PROGRAM PickAndPlace //TF5420 PickAndPlace解决方案
VAR	
	(*抓取动作功能块（其中重要的以***标出）*)
	//轴组相关功能块
    fbAddAllAxes			                     : FB_AddAllAxes;//***将笛卡尔坐标系轴加入组
	fbGroupEnable			                     : MC_GroupEnable;//***轴组使能
	fbStop					                     : MC_GroupStop;//轴组停止
	fbUngroupAxes			                     : MC_UngroupAllAxes;//解耦轴组
	fbGroupReset			                     : MC_GroupReset;//***轴组复位
	fbGroupReadStatus		                     : MC_GroupReadStatus;//***读取轴组状态,用于报错判断
	fbGroupSetOvr			                     : MC_GroupSetOverride;//设定轴组override
    fbRemoveAllAxes                              : FB_RemoveAllAxes;//清除组中的所有轴
	
	//抓取、皮带跟随功能块
    fbMovePath				                     : MC_MovePath;//***插补动作与皮带跟随触发功能块
	fbMoveLinPrep			                     : MC_MoveLinearAbsolutePreparation;//***插补形式绝对定位
	buffer					                     : ARRAY[1..4096] OF BYTE;//插补路径点位数组
	path					                     : MC_PATH_DATA_REF(ADR(buffer), SIZEOF(buffer));
	fbTrackConveyBelt_01                         : MC_TrackConveyorBelt;//***皮带跟随功能块
	InitialObjectPos                             : ARRAY[1..4] OF MC_Lreal;//***相机读取物料点位
	
	//辅助功能块
    fbTestBeltMoveVelo                           : MC_MoveVelocity;//匀速运动
	fbTestBeltPower                              : MC_Power;//使能
    T20ms , T50ms ,TonResetDelay                 : Ton;//辅助计时器
	fbBeltReset                                  : MC_Reset;//皮带复位

   (*所用变量*)
	aTargetPos				: ARRAY[1..4] OF MC_LREAL;  //插补路径点位
	aTransitionParam		: ARRAY[1..2] OF MC_LREAL; //曲线的过渡转换参数
	MasterRefPos            : LREAL; //输料皮带当前位置
	lrDistance              : LREAL; //差值距离
    fVelFactor				: LREAL := 1.0;//速比
	nState					: INT := 0; //抓放动作Case步
    nGroupState             : UINT; //PickAndPlace轴组Case步
	bMovePrepError			: BOOL; //轴组准备报错步
	
	//轴组触发位标志位
	GroupEnable             : BOOL;	//轴组触发使能
	GroupReset				: BOOL; //轴组复位
	bpop1					: BOOL; //队列标志位
	RemoveAxes              : BOOL; //移除轴
	ReConfigAxis            : BOOL; //解耦轴组
	
	//NCI G代码回零功能块
	//NCI G代码功能块
	FB_BuildNciGroup            : CfgBuildExt3DGroup;//配置NCI通道
    FB_LoadNciProg              : ItpLoadProgEx;//加载G代码文件                 
	FB_StartGProg               : ItpStartStopEx;//启动停止
	FB_CfgReconfigGroup         : CfgReconfigGroup;//清除NCI通道
	FB_ItpResetGroup            : ItpResetEx2;//复位NCI通道
	FB_CfgReConfigAxis          : ARRAY[1..3] OF CfgReconfigAxis;//清除轴，从插补轴变回NC轴
	L_Override                  : LREAL  :=100;  //通道速比
	ProgName                    : STRING(255):='Home.nc';//G代码文件名
	Gstep                       : INT;
    uiItpState                  : UDINT; //插补通道状态返回值
	StartGProHome               : BOOL; //G代码回零触发位
	IsHoming                    : BOOL;
	
	
	
END_VAR

A_TrackConvey();//皮带跟随功能块调用
A_GroupCommand();//轴组指令
A_GProgHome();//G代码回零

CASE nState OF
0:  
	IF nGroupState=30 THEN//判断PickAndPlace轴组是否使能
	   gCurrentMaterial :=	gStmaterialNULL;//清零
	   //使用MemoryCmp来对比队列中是否有数据，有数组则允许取队列中的数组
	   IF (MEMCMP(pBuf1:= ADR(gArrayStmaterial[1]), pBuf2:=ADR(gStmaterialNULL) , n:=SIZEOF(gArrayStmaterial[1]) )<>0) THEN
		   bpop1	:=	TRUE; //标志为置位
		   nState	:=	1;			
	   END_IF
	END_IF
1:
   //若队列未在取数据，且可取标志位置位,则取
   IF NOT gbPushPopBusy AND bpop1 THEN
		  gfbPushPopStack.PopStack();
		  bpop1	:=	FALSE;
   END_IF
   //取数据，将数据赋值到变量中
   gfbPushPopStack(ArrayStmaterial:=gArrayStmaterial , PushStmaterial:= , PopStmaterial=> gCurrentMaterial, busy=>gbPushPopBusy );
  //相机发送物料坐标信息，将信息赋值到MC_TrackConveyOrBelt功能块中
   IF gCurrentMaterial.bmaterial THEN
	  InitialObjectPos[1]:=gCurrentMaterial.lrCenterX;//X轴
	  InitialObjectPos[2]:=gCurrentMaterial.lrCenterY;//Y轴
      InitialObjectPos[3]:=2;//Z轴
      InitialObjectPos[4]:=ABS(180-gCurrentMaterial.lrAngle);//C轴
	  MasterRefPos:=gCurrentMaterial.lrPhotoBeltPos;//输料皮带当前位置
      A_PreparePathPick();//调用抓取参数
	  nState := 20;
   END_IF

   
20:
   //计算输料皮带当前位置减去记录位置，当到达抓取范围内后便可抓取
   lrDistance:=BeltAxis.NcToPlc.ActPos-MasterRefPos  + InitialObjectPos[1];
   //抓取范围在X轴的-180到100之间，此单位内允许抓取
   IF lrDistance>=-180 AND lrDistance<=100  THEN
	    fbTrackConveyBelt_01.Execute :=TRUE;
	    IF fbTrackConveyBelt_01.Active THEN
	       nState :=220;  
	    END_IF
	ELSE //超出100的范围则判断来不及抓取，因此不抓取，返回第0步判断下一个物料
		IF lrDistance>100 THEN
		   bpop1		:= TRUE;
		   nState 		:= 0;
		END_IF
   END_IF		

220:
    //触发MC_MoveLinearAbsolutePreparation和MC_TrackConveyOrBelt
    fbMovePath.Execute:=TRUE;
	//Insync引脚和Done引脚互锁，若置位则代表机器人已经完成了物料跟踪，可以进行抓取
	IF fbTrackConveyBelt_01.InSync  AND  fbMovePath.Done  THEN
		PickorPlace:=1;//气阀吸合
	    nState := 225;  
    END_IF
225:
     //延时50ms
     T50ms(IN:= TRUE, PT:=T#1MS , Q=> , ET=> );
     //50MS后复位功能块触发位 
	 IF T50ms.Q THEN
		fbMovePath(AxesGroup:= stGroupRef, PathData:= path, Execute:= FALSE);
		fbTrackConveyBelt_01.Execute :=FALSE;
		nState := 230; 
	    T50ms(IN:= FALSE,  ); 
	 END_IF

 230:
     //触发轴组停止
	 fbStop.Execute:=TRUE;
	 //机器人停止后，复位触发位，调用放置参数
     IF fbStop.Done THEN
		nState := 240; 
		fbStop.Execute:= FALSE;
		A_PreparePathPlace();//放置参数
	 END_IF


240:
    //再次触发MC_MoveLinearAbsolutePreparation，进行物料的放置
	fbMovePath.Execute:=TRUE;
	IF  fbMovePath.Done  AND AllowtoPlace THEN //放置完成且旋切的允许放置标志位互锁，置位气阀关闭物料下降
		fbMovePath(AxesGroup:= stGroupRef, PathData:= path, Execute:= FALSE);
		PickorPlace:=0;//气阀关闭
		CutterNum:=MaterialNum;//将物料个数赋值给旋切物料个数便于后续的送料皮带启停的判断
	    MasterCutterRef:=Cutter_Master.NcToPlc.ActPos;//记录放置物料时送料皮带的当前位置
		//1号队列存取皮带当前位置，用于触发旋切时的距离判断
		gfbPushPopCutter1(ArrayCutterEnc:=gArrayCutterEnc1 , PushCutterEnc:=MasterCutterRef , PopCutterEnc=> , busy=>gbPushPopCutterBusy1 );
		gfbPushPopCutter1.PushStack();
		//2号队列存取皮带当前位置，用于皮带启停的距离判断
		gfbPushPopCutter2(ArrayCutterEnc:=gArrayCutterEnc2 , PushCutterEnc:=MasterCutterRef , PopCutterEnc=> , busy=>gbPushPopCutterBusy2 );
		gfbPushPopCutter2.PushStack();
		bpop1	:= TRUE;
		nState 	:= 250; 
	END_IF	
	
250:
    //物料个数自加
    MaterialNum:=MaterialNum+1;
	//允许放置标志位复位
    AllowtoPlace:=FALSE;
	nstate:=0;
END_CASE

ACTION A_GProgHome:
(*NCI通道状态，通常用作标志位,uiItpState返回值代表着当前插补通道的状态，其中几个重要的状态：
  1：ITP_STATE_IDLE     该状态未加载任何G代码程序或是刚执行完复位功能，插补通道处于空闲状态。若当前执行G代码停止也会进入该状态。
  2: ITP_STATE_READY    成功导入G代码程序，插补通道进入准备状态。当G代码程序被完整执行完，插补通道也会进入该状态
  5: ITP_STATE_RUNNING  正在运行G代码
 12: ITP_STATE_ABORTED  如果在G代码运行过程中出现报错，插补通道立即进入该模式，当前报错代码也会出现在通道状态中*)
uiItpState	:=	ItpGetStateInterpreter( stKinToPlc);
(*设置NCI通道的override*)
ItpSetOverridePercent(fOverridePercent:=L_Override, sPlcToNci:=stPlcToKin);

//配置插补通道功能块，设定XYZ插补轴
FB_BuildNciGroup(
	bExecute:= , 
	nGroupId:=13 , 
	nXAxisId:=AxisArray[5].NcToPlc.AxisId , 
	nYAxisId:=AxisArray[6].NcToPlc.AxisId , 
	nZAxisId:=AxisArray[7].NcToPlc.AxisId, 
	nQ1AxisId:=0 , 
	nQ2AxisId:=0 , 
	nQ3AxisId:=0 , 
	nQ4AxisId:=0 , 
	nQ5AxisId:=0, 
	tTimeOut:=T#300MS ,  );

//上载G代码功能块 
FB_LoadNciProg(
	sNciToPlc:=stKinToPlc , 
	bExecute:= , 
	sPrg:=ProgName , 
	nLength:=INT_TO_UDINT(Len(ProgName)), 
	tTimeOut:=T#300MS , );

//运行G代码功能块	
FB_StartGProg(
	bStart:= , 
	bStop:= , 
	tTimeOut:= , 
	sNciToPlc:=stKinToPlc , 
	bBusy=> , 
	bErr=> , 
	nErrId=> );

//清除插补通道功能块	
FB_CfgReconfigGroup(
	bExecute:= , 
	nGroupId:=13 , 
	tTimeOut:=T#300MS , );

FB_CfgReConfigAxis[1](
	bExecute:=ReConfigAxis , 
	nAxisId:=5 , 
	tTimeOut:=T#300MS , 
	);

FB_CfgReConfigAxis[2](
	bExecute:=ReConfigAxis , 
	nAxisId:=6 , 
	tTimeOut:=T#300MS , 
	);

FB_CfgReConfigAxis[3](
	bExecute:=ReConfigAxis , 
	nAxisId:=7 , 
	tTimeOut:=T#300MS , 
	);


//复位插补通道功能块	
FB_ItpResetGroup(
	bExecute:= , 
	tTimeOut:=T#300MS , 
	sNciToPlc:=stKinToPlc ,  );

	
	
CASE Gstep OF
0://初始化步，复位标志位及触发位
  FB_BuildNciGroup.bExecute:=FALSE;
  FB_LoadNciProg.bExecute:=FALSE;
  FB_CfgReconfigGroup.bExecute:=FALSE;
  FB_StartGProg.bStart:=FALSE;
  FB_StartGProg.bStop:=FALSE;
  ReConfigAxis:=FALSE;
  IsHoming:=FALSE;//是否正在回零标志位
  //Gstep:=10; 
  IF StartGProHome=TRUE THEN
	 Gstep:=10; 
  END_IF

10: 
  FB_BuildNciGroup.bExecute:=TRUE;
  IsHoming:=TRUE; //正在回零
  IF uiItpState=1 OR uiItpState= 2 THEN//判断NCI通道状态，初次执行时返回值为1，后续执行返回值为2
 	 Gstep:=20;
  END_IF
  IF FB_BuildNciGroup.bErr OR uiItpState= 12 THEN//报错判断步功能块报错或插补通道报错,后续报错判断步都为如此
	 Gstep:=99;
  END_IF
  
20: 
  FB_LoadNciProg.bExecute:=TRUE;
  IF  uiItpState=2 THEN  //上载G代码文件后NCI通道状态为2 
	  Gstep:=30;
  END_IF
  IF FB_LoadNciProg.bErr OR uiItpState= 12 THEN 
	 Gstep:=99;
  END_IF
 
30:
  FB_StartGProg.bStart:=TRUE; //运行G代码文件进行回零
  IF uiItpState=5 THEN  //正在运行时NCI通道状态为5
     Gstep:=40;
  END_IF
  IF FB_StartGProg.bErr OR uiItpState= 12 THEN 
	 Gstep:=99;
  END_IF

40:
  IF NOT FB_StartGProg.bBusy AND  uiItpState=2 THEN //等待是否执行完成
     StartGProHome:=FALSE;
	 FB_CfgReconfigGroup.bExecute:=TRUE; //执行完成后必须清楚NCI通道，否则与抓取程序的配置冲突
	 Gstep:=50;
  END_IF
  IF FB_CfgReconfigGroup.bErr OR uiItpState= 12 THEN 
	 Gstep:=99;
  END_IF
  
50: 
   IF NOT FB_CfgReConfigGroup.bBusy THEN 
	      ReConfigAxis:=TRUE;
		  Gstep:=0;
   END_IF
   
  
99://报错处理步,复位NCI通道并返回初始步 
  StartGProHome:=FALSE;
  FB_ItpResetGroup.bExecute:=TRUE;
  IF NOT FB_ItpResetGroup.bBusy THEN
	 Gstep:=0; 
  END_IF
END_CASE
END_ACTION

ACTION A_GroupCommand:
(*轴组使能、报错判断、复位等操作*)
//轴组状态报错判断
fbGroupReadStatus(
	AxesGroup:= stGroupRef , 
	Enable:= TRUE , 
	Valid=> , 
	Busy=> , 
	GroupMoving=> , 
	GroupHoming=> , 
	GroupErrorStop=> , 
	GroupNotReady=> , 
	GroupStandby=> , 
	GroupStopping=> , 
	GroupDisabled=> , 
	Error=> , 
	ErrorId=> );
IF fbGroupReadStatus.Error THEN
	nState := 9998;
ELSIF NOT fbGroupReadStatus.Valid THEN
	nState := 9999;	
END_IF
//定义触发功能块
fbMovePath(
		AxesGroup:=stGroupRef , 
		PathData:= path , 
		Execute:=
);
//设置轴组速比
fbGroupSetOvr(
	AxesGroup:= stGroupRef, 
	Enable:= TRUE, 
	VelFactor:= fVelFactor , 
	Enabled=> , 
	Busy=> , 
	Error=> , 
	ErrorId=> , 
	ActualVelFactor=> );
IF fbGroupSetOvr.Error THEN
   nState := 9999;
END_IF

//测试轴指令
fbTestBeltPower(
	Axis:=BeltAxis , 
	Enable:=TRUE , 
	Enable_Positive:=1 , 
	Enable_Negative:=1 , 
	Override:=100 , 
);
fbTestBeltMoveVelo(
	Axis:=BeltAxis , 
	Execute:= , 
	Velocity:=70 , 
 );
//读取皮带轴状态
beltAxis.ReadStatus();	
//轴组复位
fbBeltReset(Axis:=BeltAxis , Execute:=GroupReset ,  );

//解耦指令
fbUngroupAxes(
	AxesGroup:= stGroupRef , 
	Execute:= , 
	Done=> , 
	Busy=> , 
	Error=> , 
	ErrorId=> 
);

//轴组复位
fbGroupReset(
	AxesGroup:= stGroupRef , 
	Execute:=GroupReset , 
	Done=> , 
	Busy=> , 
	Error=> , 
	ErrorId=> );	
	
//移出轴
fbRemoveAllAxes(Execute:=RemoveAxes , Done=> , Busy=> , Error=> );

//轴组停止
fbStop(
       AxesGroup:=stGroupRef, 
       Execute:=,
      );

//加入轴组、轴组使能(轴组逻辑）
CASE nGroupState OF
0:	
    //若GroupEnable置位则运行轴组逻辑
    IF  GroupEnable THEN	
	    fbGroupEnable(AxesGroup:=stGroupRef , Execute:=FALSE);
	    fbMovePath(AxesGroup:=stGroupRef ,PathData:=path ,Execute:= FALSE);
		fbAddAllAxes(Execute:= FALSE);
		fbTestBeltMoveVelo.Execute:=FALSE;
	    bMovePrepError := FALSE;
	    nGroupState := 10;
	END_IF

10: 
	fbAddAllAxes(Execute:= TRUE);			//将所有轴都加入轴组
	fbTestBeltMoveVelo.Execute:=TRUE;       //使能虚轴
	IF fbAddAllAxes.Done  THEN				//加入轴组完成标志位
	   IF  GroupEnable THEN
		   nGroupState := 20;
	   END_IF
	ELSIF fbAddAllAxes.Error THEN			
		  nGroupState := nGroupState+1000;
	END_IF
	
20:	
	fbGroupEnable(AxesGroup:=stGroupRef , Execute:=TRUE);  //使能轴组.
	IF fbGroupEnable.Done THEN								//使能轴组完成标志位
	   fbGroupEnable(AxesGroup:=stGroupRef , Execute:=FALSE);  //复位使能轴组功能块
	   nGroupState := 30;
	ELSIF fbGroupEnable.Error THEN
		  nGroupState := nGroupState+1000;
	END_IF

30:	
	fbUngroupAxes(AxesGroup:= stGroupRef, Execute:= FALSE);  //解绑轴组结构配置
	IF  NOT GroupEnable THEN
		    nGroupState := 40;
	END_IF	
	
40:	
	fbUngroupAxes.Execute:=TRUE;				//解绑轴组
	IF fbUngroupAxes.Done THEN					//解绑轴组完成标志位
	   fbUngroupAxes.Execute:=FALSE;			//解绑轴组完成标志位
	   nGroupState:=0;
	ELSIF fbUngroupAxes.Error THEN
		  nGroupState := nGroupState+1000;
	END_IF
	
1000..9999:
IF  GroupReset THEN
	nState:=0;
	fbMovePath(AxesGroup:= stGroupRef, PathData:= path, Execute:= FALSE);
  	fbGroupEnable(AxesGroup:=stGroupRef , Execute:=FALSE);
    fbTrackConveyBelt_01.Execute:=FALSE;
	fbUngroupAxes(AxesGroup:= stGroupRef, Execute:= TRUE);
    TonResetDelay(IN:=TRUE , PT:=T#20MS, Q=> , ET=> );
END_IF
IF  TonResetDelay.Q THEN
    fbUngroupAxes(AxesGroup:= stGroupRef, Execute:= FALSE);
    TonResetDelay(IN:=FALSE , PT:=T#20MS, Q=> , ET=> );
	nGroupState:=0;
END_IF	
END_CASE
END_ACTION

ACTION A_PreparePathPick:
(*定义抓取插补路径*)

path.ClearPath();  //Clear nodes that were in path

fbMoveLinPrep.Position						:= ADR(aTargetPos); //pointer to position array
fbMoveLinPrep.PositionCount 				:= 4; //number of axes in group
fbMoveLinPrep.TransitionParameter			:= ADR (aTransitionParam); //pointer to transition parameter array
fbMoveLinPrep.TransitionParameterCount		:= 2; //number of transition parameters, has to be set always 2
fbMoveLinPrep.BufferMode					:= mcBlendingPrevious;
fbMoveLinPrep.TransitionMode				:= mcTransModeCornerDistanceAdvanced;
//Set dynamics to default values of the axes
fbMoveLinPrep.Acceleration					:= 40000;
fbMoveLinPrep.Deceleration					:= 40000;
fbMoveLinPrep.Jerk							:= 150000;

//1st node
aTargetPos[1]				:= 0;
aTargetPos[2]				:=0;
aTargetPos[3]				:= 0;
aTargetPos[4]				:= 0;
aTransitionParam[1]			:= 0; //blending distance on previous segment, no influence here
aTransitionParam[2]			:= 0; //blending distance on this segment, no influence here
fbMoveLinPrep(PathData:= path , Velocity:=1000, InvokeId:= 10);
bMovePrepError := bMovePrepError OR fbMoveLinPrep.Error;

aTargetPos[1]				:= 0;
aTargetPos[2]				:= 0;
aTargetPos[3]				:=-15;
aTargetPos[4]				:= 0;
aTransitionParam[1]			:= 45; //blending distance on previous segment (InvokeId=10), defines when to leave line
aTransitionParam[2]			:= 90;//blending distance on this segment, defines latest positionn to be back  on line of InovkeId=20 
fbMoveLinPrep(PathData:= path , Velocity:= 1000, InvokeId:= 20); 
bMovePrepError := bMovePrepError OR fbMoveLinPrep.Error;

(*aTargetPos[1]				:= 0;
aTargetPos[2]				:= 0;
aTargetPos[3]				:= 0;
aTargetPos[4]				:= 0;
aTransitionParam[1]			:= 45; 
aTransitionParam[2]			:= 85;
fbMoveLinPrep(PathData:= path , Velocity:= 400, InvokeId:= 30);
bMovePrepError := bMovePrepError OR fbMoveLinPrep.Error;*)
END_ACTION

ACTION A_PreparePathPlace:
(*定义放置插补路径*)

path.ClearPath(); //Clear nodes that were in path

fbMoveLinPrep.Position						:= ADR(aTargetPos); //pointer to position array
fbMoveLinPrep.PositionCount 				:= 4; //number of axes in group
fbMoveLinPrep.TransitionParameter			:= ADR (aTransitionParam); //pointer to transition parameter array
fbMoveLinPrep.TransitionParameterCount		:= 2; //number of transition parameters, has to be set always 2
fbMoveLinPrep.BufferMode					:= mcBlendingPrevious;
fbMoveLinPrep.TransitionMode				:= mcTransModeCornerDistanceAdvanced;
fbMoveLinPrep.Acceleration					:= 40000;
fbMoveLinPrep.Deceleration					:= 40000;
fbMoveLinPrep.Jerk							:= 150000;

aTargetPos[1]				:= 0;
aTargetPos[2]				:= -100;
aTargetPos[3]				:= 0;
aTargetPos[4]				:= 0;
aTransitionParam[1]			:= 0; //blending distance on previous segment, no influence here
aTransitionParam[2]			:= 0; //blending distance on this segment, no influence here
fbMoveLinPrep(PathData:= path , Velocity:= 1000, InvokeId:= 15);
bMovePrepError := bMovePrepError OR fbMoveLinPrep.Error; 

aTargetPos[1]				:= 0;
aTargetPos[2]				:= 0;
aTargetPos[3]				:= 0;
aTargetPos[4]				:= 0;
aTransitionParam[1]			:= 45; //blending distance on previous segment (InvokeId=10), defines when to leave line
aTransitionParam[2]			:= 90; //blending distance on this segment, defines latest positionn to be back  on line of InovkeId=20
fbMoveLinPrep(PathData:= path , Velocity:= 1000, InvokeId:= 25);
bMovePrepError := bMovePrepError OR fbMoveLinPrep.Error;

aTargetPos[1]				:= 0;
aTargetPos[2]				:= 100;
aTargetPos[3]				:= -8;
aTargetPos[4]				:= 0;
aTransitionParam[1]			:= 45; 
aTransitionParam[2]			:= 90;
fbMoveLinPrep(PathData:= path , Velocity:=700, InvokeId:= 35);
bMovePrepError := bMovePrepError OR fbMoveLinPrep.Error;
END_ACTION

ACTION A_TrackConvey:
(*皮带跟随功能块定义*)
fbTrackConveyBelt_01(
	AxesGroup:=stGroupRef , 
	ConveyorBelt:=BeltAxis , 
	Execute:= , 
	CoordTransform:=oidConveryorbelt , 
	InitialObjectPos:=ADR(InitialObjectPos) , 
	InitialObjectPosCount:=SIZEOF(InitialObjectPos)/SIZEOF(InitialObjectPos[1]) , 
	MasterRefPos:=MasterRefPos, 
	Velocity:=1000 , 
	Acceleration:=40000 , 
	Deceleration:=40000 , 
	Jerk:=150000, 
 );
END_ACTION

END_PROGRAM
